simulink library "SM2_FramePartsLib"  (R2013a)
settings: Solver=ode45  StartTime=0.0  StopTime=10.0  RelTol=1e-3
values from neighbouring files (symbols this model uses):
  m = v*BEAM.rho    [FlexBeamModelConstruct2.m]    (also in FlexBeamModelConstruct3.m = BEAM.rho*v; FlexBeam_1D_Construct.m = REF.m/REF.l*a.*(linspace(1-OPT.MassBiais+1e-6,1+OPT.MassBiai; FlexBeam_3D_Construct.m = REF.m/REF.l*a.*(linspace(1-OPT.MassBiais+1e-6,1+OPT.MassBiai; FreeFlexBeam_3D_Construct.m = REF.m/REF.l*a.*tmp2)
  s = -sign(imag(KGZ_fr_tmp))    [LinprogReguliOptimFunc_1.m]    (also in LinprogReguliOptimFunc_2.m; LinprogReguliOptimFunc_1 - Copie.m)
  X = cos(phi(i))*x+sin(phi(i))*y    [MGI.m]
  Y = fft(y(:,i),NFFT)/L    [fft_bis.m]    (also in MGI.m = -sin(phi(i))*x+cos(phi(i))*y)
  Z = z    [MGI.m]
undefined symbols (not defined in the file or in its folder): kg, SimParam
libraries: sm_lib x13, nesl_utility x2

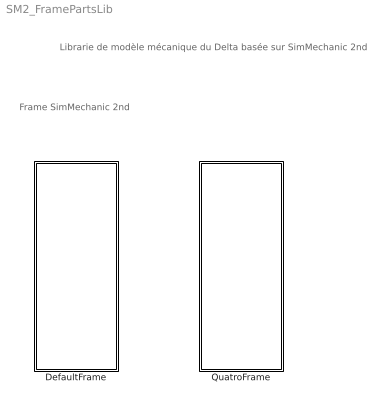
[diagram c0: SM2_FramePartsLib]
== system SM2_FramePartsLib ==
  note: Frame SimMechanic 2nd
  note: Librarie de modèle mécanique du Delta basée sur SimMechanic 2nd
  DefaultFrame : Subsystem  InitFcn=SimParam.Frame = frame_paramInitFnc(RawParam,IC);
  QuatroFrame : Subsystem  InitFcn=SimParam.Frame = frame_paramInitFnc(RawParam,IC);

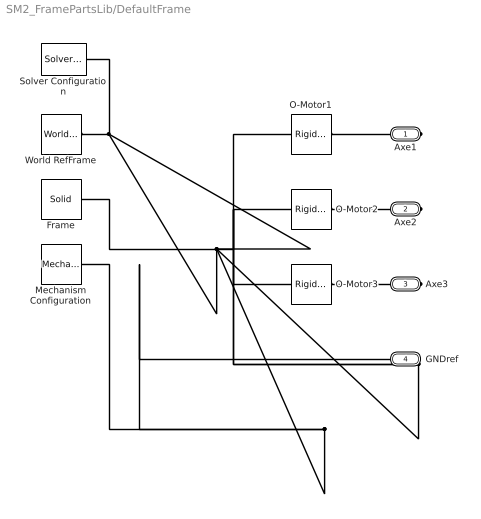
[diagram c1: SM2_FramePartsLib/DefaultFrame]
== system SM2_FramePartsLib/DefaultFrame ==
  Frame : sm_lib/Body Elements/Solid  InertiaType=CalculateFromGeometry  Mass=1  MassUnits=kg  CenterOfMass=[0 0 0]  CenterOfMassUnits=m  MomentsOfInertia=[1 1 1]  MomentsOfInertiaUnits=kg*m^2  ProductsOfInertia=[0 0 0]  ProductsOfInertiaUnits=kg*m^2  DensityBased=on  Density=1000  DensityUnits=kg/(m^3)  GraphicType=FromGeometry  MarkerShape=Sphere  MarkerSize=10  MarkerSizeUnits=m  GraphicVisPropType=SimpleVisualProperties  GraphicDiffuseColor=[0.6 0.5 0]  GraphicSpecularColor=[0.5 0.5 0.5 1.0]  GraphicAmbientColor=[0.15 0.15 0.15 1.0]  GraphicEmissiveColor=[0.0 0.0 0.0 1.0]  GraphicShininess=75  GraphicOpacity=0.5  GeometryShape=Cylinder  RectangleSize=[1 1]  RectangleSizeUnits=m  BrickDimensions=[0.3 0.3 0.001]  BrickDimensionUnits=m  CylinderRadius=SimParam.Frame.R  CylinderRadiusUnits=m  CylinderLength=0.01  CylinderLengthUnits=m  SphereRadius=1  SphereRadiusUnits=m  EllipsoidRadii=[1 1 1]  EllipsoidRadiiUnits=m  ExtrusionCrossSection=[1 1; -1 1; -1 -1; 1 -1]  ExtrusionCrossSectionUnits=m  ExtrusionLength=1  ExtrusionLengthUnits=m  PolygonNumSides=3  PolygonOuterRadius=1  PolygonOuterRadiusUnits=m  ExtGeomFileUnits=m  RevolutionCrossSection=[1 1; 1 -1; 2 -1; 2 1]  RevolutionCrossSectionUnits=m  RevolutionExtent=Full  RevolutionAngle=180  RevolutionAngleUnits=deg  BlockFunction=simmechanics.library.body_elements.solid
  Mechanism Configuration : sm_lib/Utilities/Mechanism  Configuration  GravityVector=[0 0 0]  GravityUnits=m/s^2  AllowGravitySignal=off  LinearizationDelta=0.001  BlockFunction=simmechanics.library.utilities.mechanism_configuration
  O-Motor1 : sm_lib/Frames and  Transforms/Rigid  Transform  TranslationMethod=Cylindrical  TranslationLengthUnit=m  TranslationStandardAxis=+Z  TranslationStandardOffset=0  TranslationCartesianOffset=[0 0 0]  TranslationROffset=SimParam.Frame.R  TranslationROffsetUnits=m  TranslationZOffset=0  TranslationZOffsetUnits=m  TranslationThetaOffset=SimParam.Frame.Theta(1)  TranslationThetaOffsetUnits=rad  RotationMethod=StandardAxis  RotationAngleUnits=rad  RotationStandardAxis=+Z  RotationAngle=SimParam.Frame.Theta(1)  RotationArbitraryAxis=[1,0,0]  FollAlignAxisA=+X  BaseAlignAxisA=+Y  FollAlignAxisB=+Y  BaseAlignAxisB=+Z  BlockFunction=simmechanics.library.frames_transforms.rigid_transform
  O-Motor2 : sm_lib/Frames and  Transforms/Rigid  Transform  TranslationMethod=Cylindrical  TranslationLengthUnit=m  TranslationStandardAxis=+Z  TranslationStandardOffset=0  TranslationCartesianOffset=[0 0 0]  TranslationROffset=SimParam.Frame.R  TranslationROffsetUnits=m  TranslationZOffset=0  TranslationZOffsetUnits=m  TranslationThetaOffset=SimParam.Frame.Theta(2)  TranslationThetaOffsetUnits=rad  RotationMethod=StandardAxis  RotationAngleUnits=rad  RotationStandardAxis=+Z  RotationAngle=SimParam.Frame.Theta(2)  RotationArbitraryAxis=[1,0,0]  FollAlignAxisA=+X  BaseAlignAxisA=+Y  FollAlignAxisB=+Y  BaseAlignAxisB=+Z  BlockFunction=simmechanics.library.frames_transforms.rigid_transform
  O-Motor3 : sm_lib/Frames and  Transforms/Rigid  Transform  TranslationMethod=Cylindrical  TranslationLengthUnit=m  TranslationStandardAxis=+Z  TranslationStandardOffset=0  TranslationCartesianOffset=[0 0 0]  TranslationROffset=SimParam.Frame.R  TranslationROffsetUnits=m  TranslationZOffset=0  TranslationZOffsetUnits=m  TranslationThetaOffset=SimParam.Frame.Theta(3)  TranslationThetaOffsetUnits=rad  RotationMethod=StandardAxis  RotationAngleUnits=rad  RotationStandardAxis=+Z  RotationAngle=SimParam.Frame.Theta(3)  RotationArbitraryAxis=[1,0,0]  FollAlignAxisA=+X  BaseAlignAxisA=+Y  FollAlignAxisB=+Y  BaseAlignAxisB=+Z  BlockFunction=simmechanics.library.frames_transforms.rigid_transform
  Solver Configuration : nesl_utility/Solver Configuration  PhysicalDomain=network_engine_domain  SubClassName=solver  LeftPortType=input  RightPortType=generic  Accelerate=off  Tones=[]  Harmonics=[]  SimulateNoise=off  Profile=off  UseLocalSampling=off  EnableSwitchedLinearOptims=on  FrequencyDomain=off  UseCCode=off  UseNewInitialization=off  DoDC=off  ResidualTolerance=1e-09  UseLocalSolver=off  LocalSolverChoice=NE_BACKWARD_EULER_ADVANCER  LocalSolverSampleTime=0.001  DoFixedCost=off  MaxNonlinIter=3  MaxModeIter=2  LinearAlgebra=Sparse  DelaysMemoryBudget=1024
  World RefFrame : sm_lib/Frames and  Transforms/World Frame  BlockFunction=simmechanics.library.frames_transforms.world_frame
  Axe1 : PMIOPort  Port=1  Side=Right
  Axe2 : PMIOPort  Port=2  Side=Right
  Axe3 : PMIOPort  Port=3  Side=Right
  GNDref : PMIOPort  Port=4  Side=Left
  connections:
  World RefFrame/RConn1 -- Solver Configuration/RConn1 -- O-Motor3/LConn1 -- O-Motor2/LConn1 -- O-Motor1/LConn1 -- GNDref/RConn1 -- Mechanism Configuration/RConn1 -- Frame/RConn1
  Axe3/RConn1 -- O-Motor3/RConn1
  Axe2/RConn1 -- O-Motor2/RConn1
  Axe1/RConn1 -- O-Motor1/RConn1

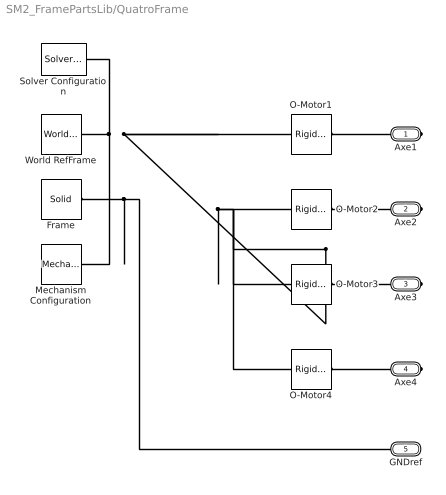
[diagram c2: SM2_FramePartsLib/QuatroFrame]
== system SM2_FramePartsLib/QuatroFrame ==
  Frame : sm_lib/Body Elements/Solid  InertiaType=CalculateFromGeometry  Mass=1  MassUnits=kg  CenterOfMass=[0 0 0]  CenterOfMassUnits=m  MomentsOfInertia=[1 1 1]  MomentsOfInertiaUnits=kg*m^2  ProductsOfInertia=[0 0 0]  ProductsOfInertiaUnits=kg*m^2  DensityBased=on  Density=1000  DensityUnits=kg/(m^3)  GraphicType=FromGeometry  MarkerShape=Sphere  MarkerSize=10  MarkerSizeUnits=m  GraphicVisPropType=SimpleVisualProperties  GraphicDiffuseColor=[0.6 0.5 0]  GraphicSpecularColor=[0.5 0.5 0.5 1.0]  GraphicAmbientColor=[0.15 0.15 0.15 1.0]  GraphicEmissiveColor=[0.0 0.0 0.0 1.0]  GraphicShininess=75  GraphicOpacity=0.5  GeometryShape=Cylinder  RectangleSize=[1 1]  RectangleSizeUnits=m  BrickDimensions=[0.3 0.3 0.001]  BrickDimensionUnits=m  CylinderRadius=SimParam.Frame.R  CylinderRadiusUnits=m  CylinderLength=0.01  CylinderLengthUnits=m  SphereRadius=1  SphereRadiusUnits=m  EllipsoidRadii=[1 1 1]  EllipsoidRadiiUnits=m  ExtrusionCrossSection=[1 1; -1 1; -1 -1; 1 -1]  ExtrusionCrossSectionUnits=m  ExtrusionLength=1  ExtrusionLengthUnits=m  PolygonNumSides=3  PolygonOuterRadius=1  PolygonOuterRadiusUnits=m  ExtGeomFileUnits=m  RevolutionCrossSection=[1 1; 1 -1; 2 -1; 2 1]  RevolutionCrossSectionUnits=m  RevolutionExtent=Full  RevolutionAngle=180  RevolutionAngleUnits=deg  BlockFunction=simmechanics.library.body_elements.solid
  Mechanism Configuration : sm_lib/Utilities/Mechanism  Configuration  GravityVector=[0 0 0]  GravityUnits=m/s^2  AllowGravitySignal=off  LinearizationDelta=0.001  BlockFunction=simmechanics.library.utilities.mechanism_configuration
  O-Motor1 : sm_lib/Frames and  Transforms/Rigid  Transform  TranslationMethod=Cylindrical  TranslationLengthUnit=m  TranslationStandardAxis=+Z  TranslationStandardOffset=0  TranslationCartesianOffset=[0 0 0]  TranslationROffset=SimParam.Frame.R  TranslationROffsetUnits=m  TranslationZOffset=0  TranslationZOffsetUnits=m  TranslationThetaOffset=SimParam.Frame.Theta(1)  TranslationThetaOffsetUnits=rad  RotationMethod=StandardAxis  RotationAngleUnits=rad  RotationStandardAxis=+Z  RotationAngle=SimParam.Frame.Theta(1)  RotationArbitraryAxis=[1,0,0]  FollAlignAxisA=+X  BaseAlignAxisA=+Y  FollAlignAxisB=+Y  BaseAlignAxisB=+Z  BlockFunction=simmechanics.library.frames_transforms.rigid_transform
  O-Motor2 : sm_lib/Frames and  Transforms/Rigid  Transform  TranslationMethod=Cylindrical  TranslationLengthUnit=m  TranslationStandardAxis=+Z  TranslationStandardOffset=0  TranslationCartesianOffset=[0 0 0]  TranslationROffset=SimParam.Frame.R  TranslationROffsetUnits=m  TranslationZOffset=0  TranslationZOffsetUnits=m  TranslationThetaOffset=SimParam.Frame.Theta(2)  TranslationThetaOffsetUnits=rad  RotationMethod=StandardAxis  RotationAngleUnits=rad  RotationStandardAxis=+Z  RotationAngle=SimParam.Frame.Theta(2)  RotationArbitraryAxis=[1,0,0]  FollAlignAxisA=+X  BaseAlignAxisA=+Y  FollAlignAxisB=+Y  BaseAlignAxisB=+Z  BlockFunction=simmechanics.library.frames_transforms.rigid_transform
  O-Motor3 : sm_lib/Frames and  Transforms/Rigid  Transform  TranslationMethod=Cylindrical  TranslationLengthUnit=m  TranslationStandardAxis=+Z  TranslationStandardOffset=0  TranslationCartesianOffset=[0 0 0]  TranslationROffset=SimParam.Frame.R  TranslationROffsetUnits=m  TranslationZOffset=0  TranslationZOffsetUnits=m  TranslationThetaOffset=SimParam.Frame.Theta(3)  TranslationThetaOffsetUnits=rad  RotationMethod=StandardAxis  RotationAngleUnits=rad  RotationStandardAxis=+Z  RotationAngle=SimParam.Frame.Theta(3)  RotationArbitraryAxis=[1,0,0]  FollAlignAxisA=+X  BaseAlignAxisA=+Y  FollAlignAxisB=+Y  BaseAlignAxisB=+Z  BlockFunction=simmechanics.library.frames_transforms.rigid_transform
  O-Motor4 : sm_lib/Frames and  Transforms/Rigid  Transform  TranslationMethod=Cylindrical  TranslationLengthUnit=m  TranslationStandardAxis=+Z  TranslationStandardOffset=0  TranslationCartesianOffset=[0 0 0]  TranslationROffset=SimParam.Frame.R  TranslationROffsetUnits=m  TranslationZOffset=0  TranslationZOffsetUnits=m  TranslationThetaOffset=SimParam.Frame.Theta(4)  TranslationThetaOffsetUnits=rad  RotationMethod=StandardAxis  RotationAngleUnits=rad  RotationStandardAxis=+Z  RotationAngle=SimParam.Frame.Theta(4)  RotationArbitraryAxis=[1,0,0]  FollAlignAxisA=+X  BaseAlignAxisA=+Y  FollAlignAxisB=+Y  BaseAlignAxisB=+Z  BlockFunction=simmechanics.library.frames_transforms.rigid_transform
  Solver Configuration : nesl_utility/Solver Configuration  PhysicalDomain=network_engine_domain  SubClassName=solver  LeftPortType=input  RightPortType=generic  Accelerate=off  Tones=[]  Harmonics=[]  SimulateNoise=off  Profile=off  UseLocalSampling=off  EnableSwitchedLinearOptims=on  FrequencyDomain=off  UseCCode=off  UseNewInitialization=off  DoDC=off  ResidualTolerance=1e-09  UseLocalSolver=off  LocalSolverChoice=NE_BACKWARD_EULER_ADVANCER  LocalSolverSampleTime=0.001  DoFixedCost=off  MaxNonlinIter=3  MaxModeIter=2  LinearAlgebra=Sparse  DelaysMemoryBudget=1024
  World RefFrame : sm_lib/Frames and  Transforms/World Frame  BlockFunction=simmechanics.library.frames_transforms.world_frame
  Axe1 : PMIOPort  Port=1  Side=Right
  Axe2 : PMIOPort  Port=2  Side=Right
  Axe3 : PMIOPort  Port=3  Side=Right
  Axe4 : PMIOPort  Port=4  Side=Right
  GNDref : PMIOPort  Port=5  Side=Left
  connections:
  Axe1/RConn1 -- O-Motor1/RConn1
  Axe2/RConn1 -- O-Motor2/RConn1
  Axe3/RConn1 -- O-Motor3/RConn1
  Frame/RConn1 -- Mechanism Configuration/RConn1 -- GNDref/RConn1 -- O-Motor1/LConn1 -- O-Motor4/LConn1 -- O-Motor3/LConn1 -- O-Motor2/LConn1 -- Solver Configuration/RConn1 -- World RefFrame/RConn1
  Axe4/RConn1 -- O-Motor4/RConn1
